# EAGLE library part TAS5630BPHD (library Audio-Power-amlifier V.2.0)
300W STEREO / 600W MONO PurePath ? HD ANALOG-INPUT POWER STAGE CW07/2009
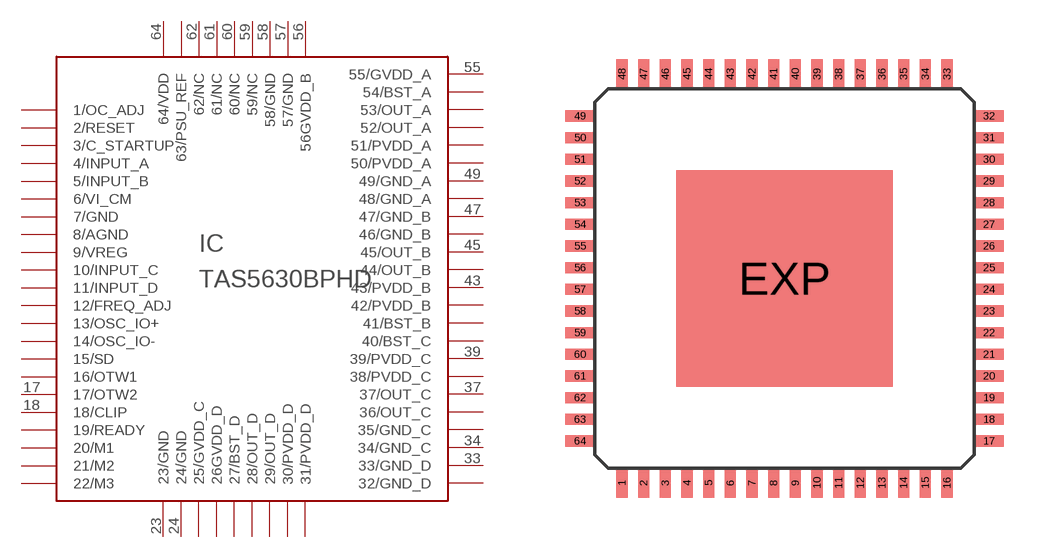
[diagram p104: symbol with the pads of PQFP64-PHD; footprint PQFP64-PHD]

Designator prefix IC

## TAS5630BPHDTAS5630BPHD  [PQFP64-PHD]
1  1/OC_ADJ
2  2/RESET  in
3  3/C_STARTUP
4  4/INPUT_A  in
5  5/INPUT_B  in
6  6/VI_CM
7  7/GND  pwr
8  8/AGND  pwr
9  9/VREG
10  10/INPUT_C  in
11  11/INPUT_D  in
12  12/FREQ_ADJ
13  13/OSC_IO+
14  14/OSC_IO-
15  15/SD  out
16  16/OTW1  out
17  17/OTW2
18  18/CLIP
19  19/READY
20  20/M1
21  21/M2
22  22/M3
23  23/GND  pwr
24  24/GND  pwr
25  25/GVDD_C
26  26GVDD_D
27  27/BST_D
28  28/OUT_D
29  29/OUT_D
30  30/PVDD_D
31  31/PVDD_D
32  32/GND_D  pwr
33  33/GND_D  pwr
34  34/GND_C  pwr
35  35/GND_C  pwr
36  36/OUT_C  out
37  37/OUT_C  out
38  38/PVDD_C
39  39/PVDD_C
40  40/BST_C
41  41/BST_B
42  42/PVDD_B
43  43/PVDD_B
44  44/OUT_B  out
45  45/OUT_B  out
46  46/GND_B  pwr
47  47/GND_B  pwr
48  48/GND_A  pwr
49  49/GND_A  pwr
50  50/PVDD_A
51  51/PVDD_A
52  52/OUT_A  out
53  53/OUT_A  out
54  54/BST_A
55  55/GVDD_A
56  56GVDD_B
57  57/GND  pwr
58  58/GND  pwr
59  59/NC  nc
60  60/NC  nc
61  61/NC  nc
62  62/NC  nc
63  63/PSU_REF
64  64/VDD  pwr

## Footprint PQFP64-PHD (pad centres in mm)
64-Pin QFP (PHD) power package
smd 0.41 x 1.1: 1 -6,-7.55; 2 -5.2,-7.55; 3 -4.4,-7.55; 4 -3.6,-7.55; 5 -2.8,-7.55; 6 -2,-7.55; 7 -1.2,-7.55; 8 -0.4,-7.55; 9 0.4,-7.55; 10 1.2,-7.55; 11 2,-7.55; 12 2.8,-7.55; 13 3.6,-7.55; 14 4.4,-7.55; 15 5.2,-7.55; 16 6,-7.55; 33 6,7.55; 34 5.2,7.55; 35 4.4,7.55; 36 3.6,7.55; 37 2.8,7.55; 38 2,7.55; 39 1.2,7.55; 40 0.4,7.55; 41 -0.4,7.55; 42 -1.2,7.55; 43 -2,7.55; 44 -2.8,7.55; 45 -3.6,7.55; 46 -4.4,7.55; 47 -5.2,7.55; 48 -6,7.55
smd 1.1 x 0.41: 17 7.55,-6; 18 7.55,-5.2; 19 7.55,-4.4; 20 7.55,-3.6; 21 7.55,-2.8; 22 7.55,-2; 23 7.55,-1.2; 24 7.55,-0.4; 25 7.55,0.4; 26 7.55,1.2; 27 7.55,2; 28 7.55,2.8; 29 7.55,3.6; 30 7.55,4.4; 31 7.55,5.2; 32 7.55,6; 49 -7.55,6; 50 -7.55,5.2; 51 -7.55,4.4; 52 -7.55,3.6; 53 -7.55,2.8; 54 -7.55,2; 55 -7.55,1.2; 56 -7.55,0.4; 57 -7.55,-0.4; 58 -7.55,-1.2; 59 -7.55,-2; 60 -7.55,-2.8; 61 -7.55,-3.6; 62 -7.55,-4.4; 63 -7.55,-5.2; 64 -7.55,-6
smd 8 x 8: EXP 0,0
